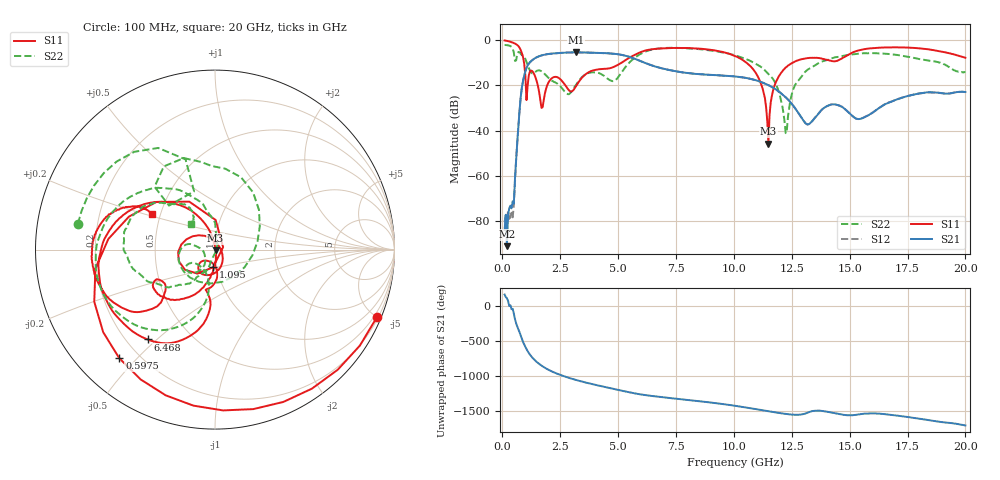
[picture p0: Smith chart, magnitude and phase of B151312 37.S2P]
!  2-Port S-parameters saved by WinCal
! VAR MeasName=S-Parameters (CALIBRATED_DATA) read from VNA (N5244A)
! VAR MeasDate=12/8/2015 5:46:32 PM
! VAR NAME=B151312 37
! VAR FILENAME=B151312 37.S2P
! VAR DATE=12/8/2015 5:46:32 PM
! VAR PHYS_PORTS=1,2
# Hz S DB R 50
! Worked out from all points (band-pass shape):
!   401 points, 100 MHz to 20 GHz, reference 50 ohm
!   highest |S21| = -5.45 dB at 3.184 GHz (marker M1); lowest = -91.0 dB at 199.5 MHz (marker M2)
!   |S21| within 3 dB of the highest: 1.35 GHz to 5.764 GHz (4.413 GHz wide, 124 % of centre)
!   lowest |S11| = -45.8 dB at 11.49 GHz (marker M3), VSWR 1.01, Z = 50.3 - j0.379 ohm
!   |S11| at or under -10 dB: 939.3 MHz to 5.155 GHz (4.216 GHz wide, 138 % of centre); 10.54 GHz to 12.54 GHz (1.996 GHz wide, 17.3 % of centre)
!   |S22| runs from -41.2 to -2.2 dB; largest |S21 - S12| = 0.0016
!   S11 on the Smith chart (normalised r, x): 100 MHz: 0.29, -4.99; 597.5 MHz: 0.13, -0.45; 1.095 GHz: 0.96, -0.19; 6.468 GHz: 0.28, -0.47; 20 GHz: 0.45, +0.21
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1e8  -0.20 -22.6  -83.90 164.2  -80.27 -179.6  -2.19 169.3
1.995e8  -0.38 -44.4  -91.04 111.9  -81.35 74.2  -2.28 158.2
3.985e8  -0.94 -87.1  -74.34 -46.4  -76.28 -9.9  -3.02 129.5
5.975e8  -1.87 -131.3  -52.78 112.5  -52.56 113.1  -9.01 136.3
8.4625e8  -5.79 159.0  -20.94 -112.8  -20.94 -112.8  -6.63 92.3
1.095e9  -20.08 -96.3  -11.22 72.5  -11.22 72.5  -11.02 27.4
1.54275e9  -20.45 126.4  -7.36 -97.3  -7.36 -97.3  -13.44 -144.7
1.9905e9  -18.85 -79.7  -6.19 166.4  -6.18 166.4  -16.68 167.7
2.53775e9  -17.64 -134.8  -5.69 88.0  -5.68 88.0  -20.80 172.9
3.1845e9  -20.39 -88.5  -5.45 19.6  -5.44 19.6  -19.72 -124.4
3.43325e9  -16.72 -84.9  -5.48 -2.9  -5.48 -2.9  -16.47 -127.3
4.5775e9  -12.59 -101.7  -5.88 -91.6  -5.87 -91.5  -17.26 -146.7
6.468e9  -4.07 -126.9  -11.27 149.9  -11.24 149.8  -4.24 -137.2
6.7665e9  -3.78 -135.3  -12.17 138.2  -12.17 138.1  -3.74 -148.2
1.005e10  -7.04 144.0  -16.11 9.7  -16.11 9.6  -6.74 131.7
1.099525e10  -15.38 112.9  -17.91 -40.5  -17.91 -40.5  -10.84 108.5
1.149275e10  -45.83 -47.4  -19.93 -68.3  -19.92 -68.3  -15.00 95.4
1.2239e10  -12.12 -110.5  -25.29 -106.8  -25.27 -106.9  -41.15 1.5
1.2637e10  -9.51 -124.6  -30.00 -119.4  -29.95 -119.5  -19.98 -109.5
1.338325e10  -7.85 -144.5  -35.82 -66.6  -35.82 -66.9  -11.96 -130.1
1.67165e10  -3.28 -171.5  -27.56 -118.2  -27.46 -119.0  -6.20 155.8
2e10  -7.83 150.5  -22.95 87.6  -23.01 87.3  -14.24 133.4
